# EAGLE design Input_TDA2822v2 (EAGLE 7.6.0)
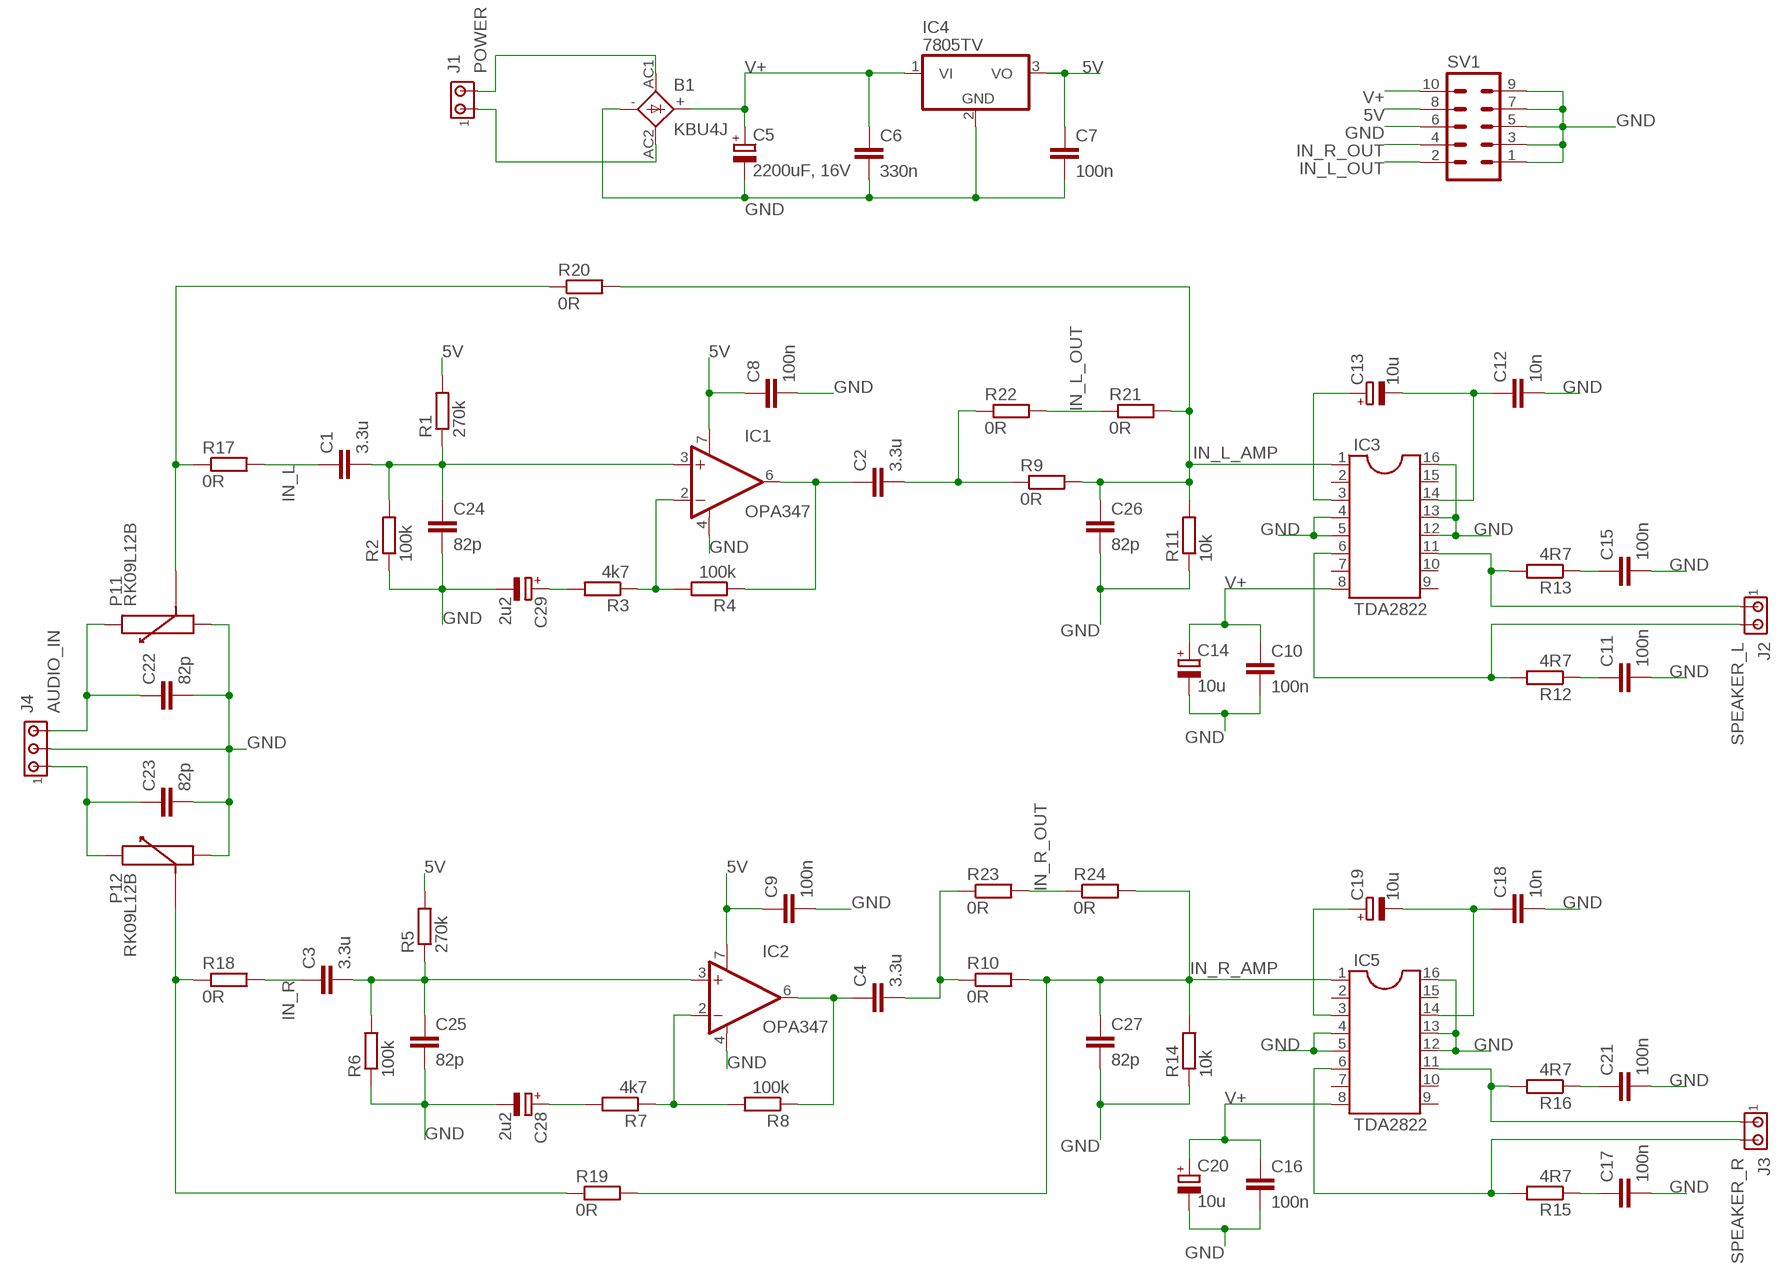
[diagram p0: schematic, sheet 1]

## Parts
B1  KBU4J  KBU  [KBU]
C1  3.3u  C-EU050-055X075  [C050-055X075]
C2  3.3u  C-EU050-055X075  [C050-055X075]
C3  3.3u  C-EU050-055X075  [C050-055X075]
C4  3.3u  C-EU050-055X075  [C050-055X075]
C5  2200uF, 16V  CPOL-EUE5-13  [E5-13]
C6  330n  C-EU050-035X075  [C050-035X075]
C7  100n  C-EU050-025X075  [C050-025X075]
C8  100n  C-EU050-025X075  [C050-025X075]
C9  100n  C-EU050-025X075  [C050-025X075]
C10  100n  C-EU050-025X075  [C050-025X075]
C11  100n  C-EU050-025X075  [C050-025X075]
C12  10n  C-EU025-025X050  [C025-025X050]
C13  10u  CPOL-EUE2-5  [E2-5]
C14  10u  CPOL-EUE2-5  [E2-5]
C15  100n  C-EU050-025X075  [C050-025X075]
C16  100n  C-EU050-025X075  [C050-025X075]
C17  100n  C-EU050-025X075  [C050-025X075]
C18  10n  C-EU025-025X050  [C025-025X050]
C19  10u  CPOL-EUE2-5  [E2-5]
C20  10u  CPOL-EUE2-5  [E2-5]
C21  100n  C-EU050-025X075  [C050-025X075]
C22  82p  C-EU025-024X044  [C025-024X044]
C23  82p  C-EU025-024X044  [C025-024X044]
C24  82p  C-EU025-024X044  [C025-024X044]
C25  82p  C-EU025-024X044  [C025-024X044]
C26  82p  C-EU025-024X044  [C025-024X044]
C27  82p  C-EU025-024X044  [C025-024X044]
C28  2u2  CPOL-EUE2-5  [E2-5]
C29  2u2  CPOL-EUE2-5  [E2-5]
IC1  OPA347  OPA336P  [DIL08]
IC2  OPA347  OPA336P  [DIL08]
IC3  TDA2822  DIL16S  [SOCKET-16]
IC4  7805TV  [TO220V]
IC5  TDA2822  DIL16S  [SOCKET-16]
J1  POWER  350428-1  [350428-1]
J2  SPEAKER_L  350428-1  [350428-1]
J3  SPEAKER_R  350428-1  [350428-1]
J4  AUDIO_IN  350429-1  [350429-1]
P1  RK09L12B  [ALPS-RK09L12B0]
R1  270k  R-EU_0309/V  [0309V]
R2  100k  R-EU_0309/V  [0309V]
R3  4k7  R-EU_0309/V  [0309V]
R4  100k  R-EU_0309/V  [0309V]
R5  270k  R-EU_0309/V  [0309V]
R6  100k  R-EU_0309/V  [0309V]
R7  4k7  R-EU_0309/V  [0309V]
R8  100k  R-EU_0309/V  [0309V]
R9  0R  R-EU_R0603  [R0603]
R10  0R  R-EU_R0603  [R0603]
R11  10k  R-EU_0309/V  [0309V]
R12  4R7  R-EU_0309/V  [0309V]
R13  4R7  R-EU_0309/V  [0309V]
R14  10k  R-EU_0309/V  [0309V]
R15  4R7  R-EU_0309/V  [0309V]
R16  4R7  R-EU_0309/V  [0309V]
R17  0R  R-EU_R0603  [R0603]
R18  0R  R-EU_R0603  [R0603]
R19  0R  R-EU_R0603  [R0603]
R20  0R  R-EU_R0603  [R0603]
R21  0R  R-EU_R0603  [R0603]
R22  0R  R-EU_R0603  [R0603]
R23  0R  R-EU_R0603  [R0603]
R24  0R  R-EU_R0603  [R0603]
SV1  ML10  [ML10]

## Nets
5V: C7.1 C8.1 C9.1 IC1.7(V+) IC2.7(V+) IC4.3(VO) R1.2 R5.2 SV1.8
GND: B1.- C5.- C6.2 C7.2 C8.2 C9.2 C10.2 C11.2 C12.2 C14.- C15.2 C16.2 C17.2 C18.2 C20.- C21.2 C22.2 C23.2 C24.2 C25.2 C26.2 C27.2 C28.- C29.- IC1.4(V-) IC2.4(V-) IC3.4 IC3.5 IC3.12 IC3.13 IC3.16 IC4.2(GND) IC5.4 IC5.5 IC5.12 IC5.13 IC5.16 J4.2 P1.GND1(1:GND$1) P1.GND2(2:GND$1) R2.1 R6.1 R11.1 R14.1 SV1.1 SV1.3 SV1.5 SV1.6 SV1.7 SV1.9
IN_L: C1.1 R17.2
IN_L_AMP: C26.1 IC3.1 R9.2 R11.2 R20.2 R21.2
IN_L_OUT: R21.1 R22.2 SV1.2
IN_R: C3.1 R18.2
IN_R_AMP: C27.1 IC5.1 R10.2 R14.2 R19.2 R24.2
IN_R_OUT: R23.2 R24.1 SV1.4
N$1: C1.2 C24.1 IC1.3(+IN) R1.1 R2.2
N$2: C3.2 C25.1 IC2.3(+IN) R5.1 R6.2
N$3: IC1.2(-IN) R3.1 R4.2
N$4: IC2.2(-IN) R7.1 R8.2
N$5: C2.1 IC1.6(OUT) R4.1
N$6: C4.1 IC2.6(OUT) R8.1
N$7: B1.AC1 J1.2
N$8: B1.AC2 J1.1
N$9: C29.+ R3.2
N$10: IC3.6 J2.2 R12.2
N$11: C28.+ R7.2
N$12: C2.2 R9.1 R22.1
N$13: C4.2 R10.1 R23.1
N$14: C19.+ IC5.3
N$15: C13.+ IC3.3
N$16: C12.1 C13.- IC3.14
N$17: C11.1 R12.1
N$18: C18.1 C19.- IC5.14
N$19: IC5.6 J3.2 R15.2
N$20: C17.1 R15.1
N$21: IC3.11 J2.1 R13.2
N$22: C15.1 R13.1
N$23: IC5.11 J3.1 R16.2
N$24: C21.1 R16.1
N$25: C22.1 J4.3 P1.IN1(1:IN$1)
N$27: C23.1 J4.1 P1.IN2(2:IN$1)
N$28: P1.OUT2(2:OUT$1) R18.1 R19.1
N$29: P1.OUT1(1:OUT$1) R17.1 R20.1
V+: B1.+ C5.+ C6.1 C10.1 C14.+ C16.1 C20.+ IC3.8 IC4.1(VI) IC5.8 SV1.10
Unconnected: IC3.2 IC3.7 IC3.9 IC3.10 IC3.15 IC5.2 IC5.7 IC5.9 IC5.10 IC5.15

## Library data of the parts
B1 = rectifier:KBU: DIOTEC RECTIFIER
C1-C4 C6-C12 C15-C18 C21-C27 = rcl:C-EU: CAPACITOR, European symbol
C5 C13 C14 C19 C20 C28 C29 = rcl:CPOL-EU: POLARIZED CAPACITOR, European symbol
IC1 IC2 = burr-brown:OPA336: CMOS Operational Amplifiers Single-Supply, MicroPower, MicroAmplifier(TM) Series; OC_FARNELL: unknown; OC_NEWARK: unknown
IC3 IC5 = ic-package:DIL16: Dual In Line / Socket
IC4 = linear:78*: Positive VOLTAGE REGULATOR Source: http://cache.national.com/ds/LM/LM78L05.pdf http://www.fairchildsemi.com/ds/LM/LM7805.pdf
J1-J3 = con-amp:350428-1: Universal MATE-N-LOK .250" Centerline, 600 V, 19 - 36 A max
J4 = con-amp:350429-1: Universal MATE-N-LOK .250" Centerline, 600 V, 19 - 36 A max Source: http://catalog.tycoelectronics.com/ .. ENG_CD_350429_Y.pdf
P1 = my:RK09L12B
R1-R24 = rcl:R-EU_: RESISTOR, European symbol
SV1 = con-ml:ML10: HARTING; OC_FARNELL: unknown; OC_NEWARK: unknown

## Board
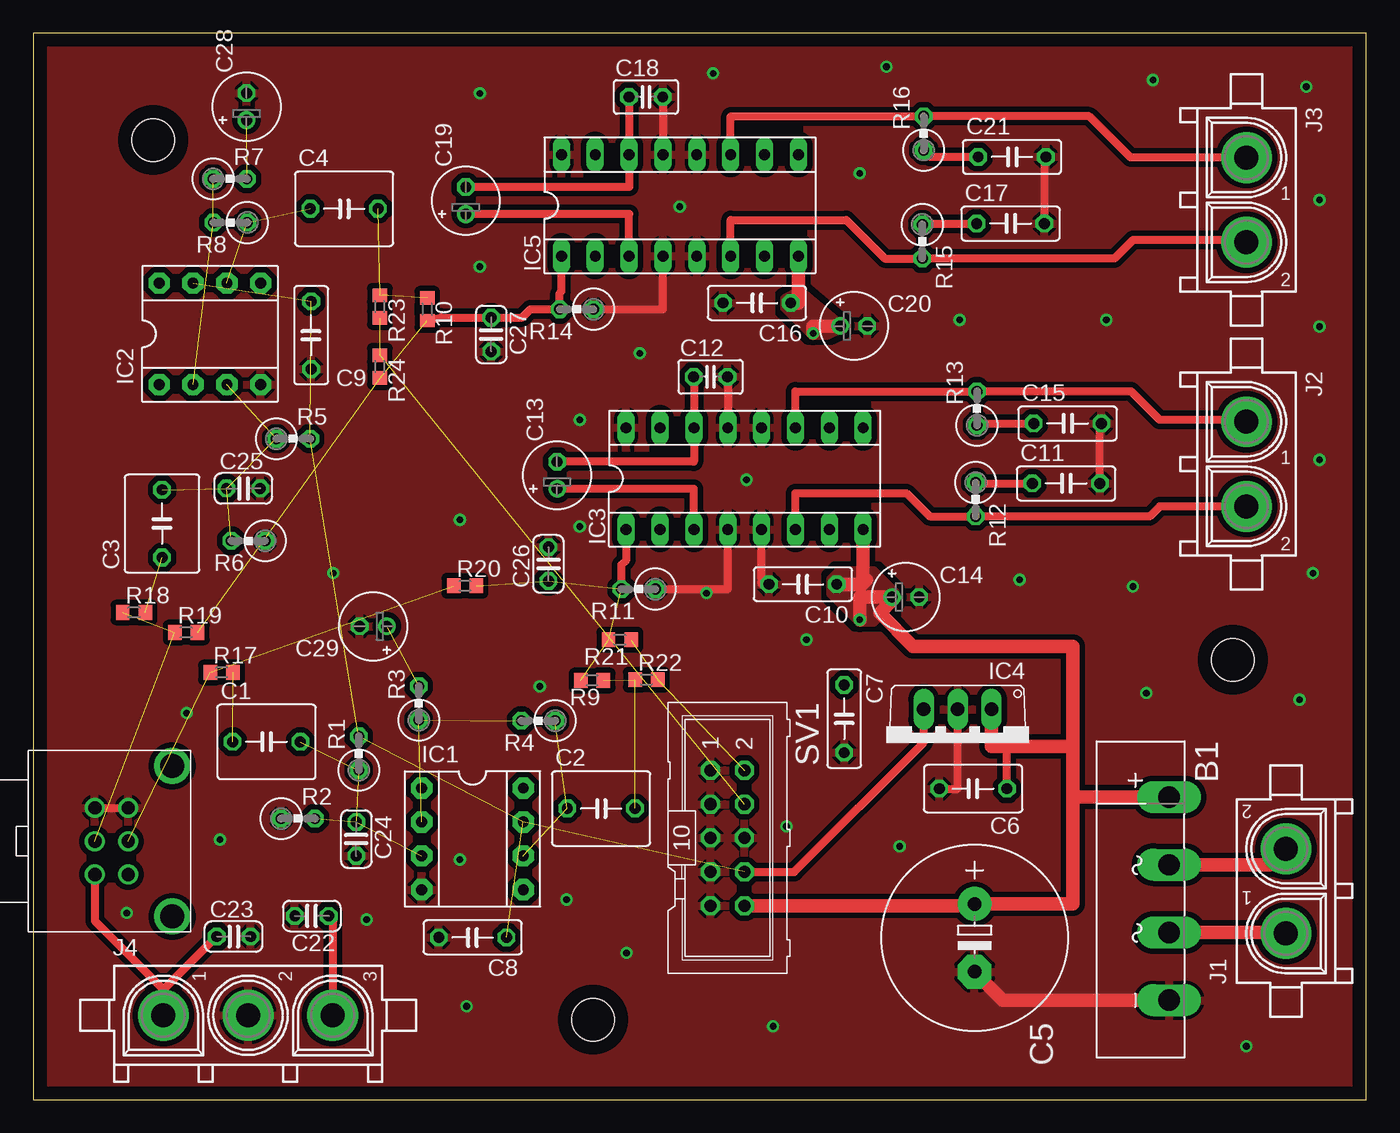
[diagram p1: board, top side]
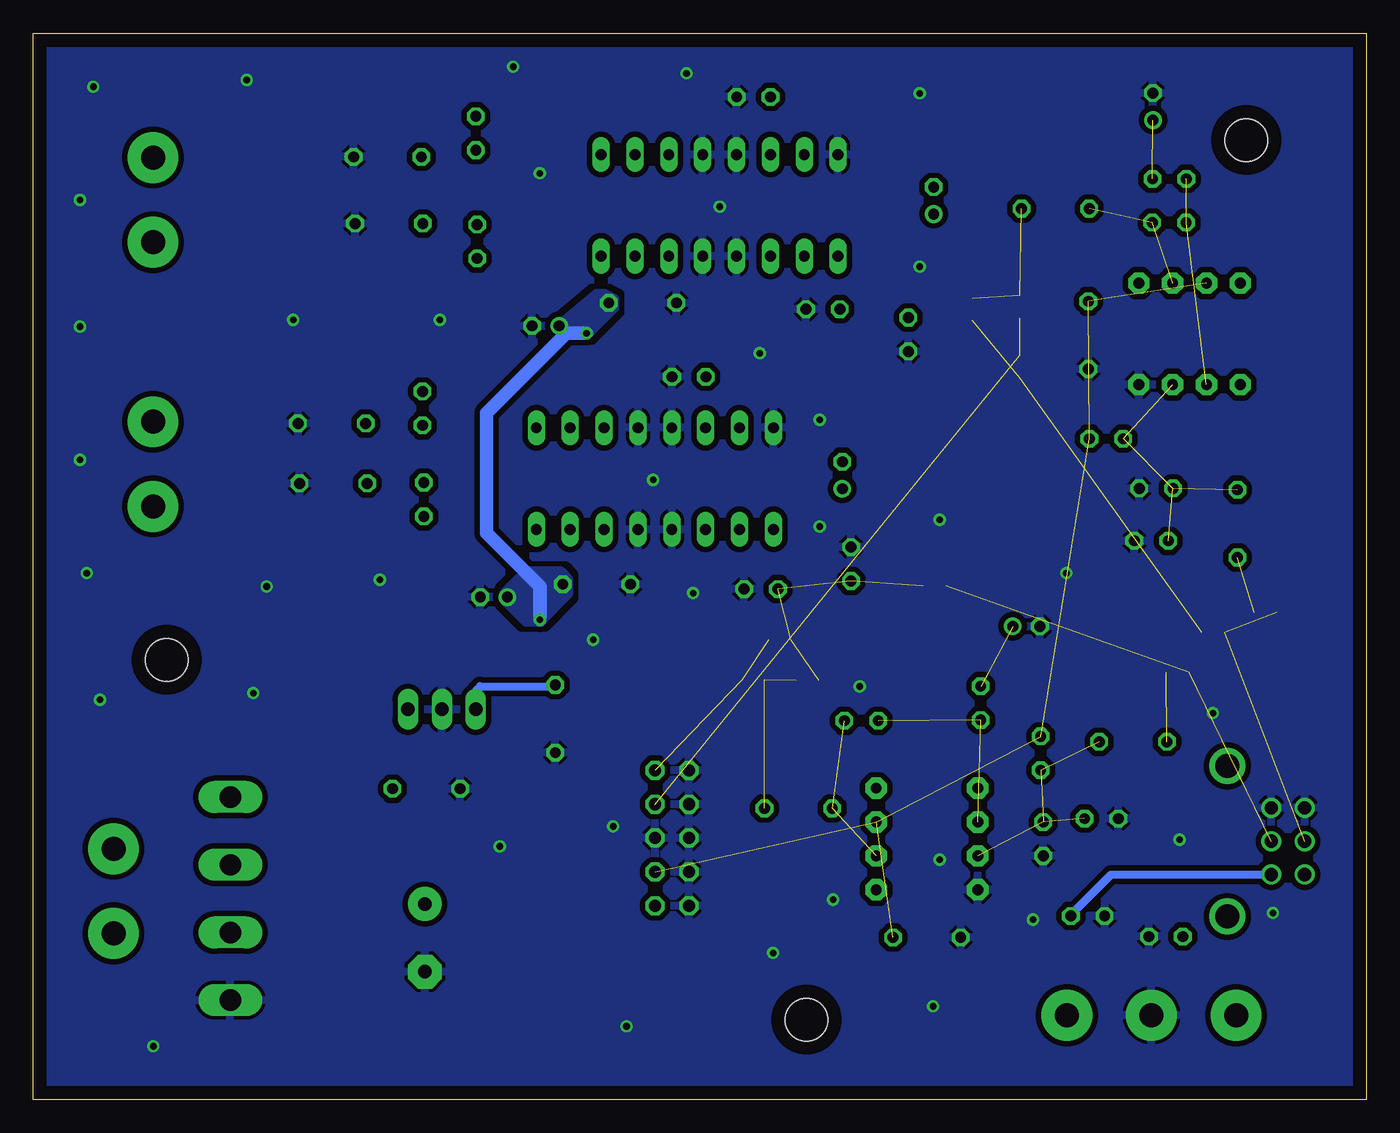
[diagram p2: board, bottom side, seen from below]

Size 100 x 80 mm. Coordinates in mm from the lower left corner, seen from the top.
Outline: 0,0 100,0 100,80 0,80 0,0
Copper layers (1*16): Top 0.035mm / dielectric 1.5mm / Bottom 0.035mm
Design rules "default": minimum track width 10mil, minimum drill 24mil, track to track 8mil, track to pad 8mil, pad to pad 8mil, via to via 8mil, smd to smd 8mil, copper to edge 40mil, drill to drill 8mil, minimum pad ring 10mil, minimum via ring 8mil, stop-mask expansion 4mil, vias tented up to drill 0mil, thermal gap 10mil
Holes 3.2 mm at 9,72 90,33 42,6

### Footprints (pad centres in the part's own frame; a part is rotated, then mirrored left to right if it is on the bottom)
KBU = drill 1.6 long: + -7.62,2.54; - 7.62,2.54; AC1 -2.54,2.54; AC2 2.54,2.54
C050-055X075 = drill 0.813 octagon: 1 -2.54,0; 2 2.54,0
E5-13 = drill 1.016 pad 2.54: + -2.54,0 | drill 1.016 pad 2.54 octagon: - 2.54,0
C050-035X075 = drill 0.813 octagon: 1 -2.54,0; 2 2.54,0
C050-025X075 = drill 0.813 octagon: 1 -2.54,0; 2 2.54,0
C025-025X050 = drill 0.813 octagon: 1 -1.27,0; 2 1.27,0
E2-5 = drill 0.813 pad 1.27: + -1.016,0 | drill 0.813 pad 1.27 octagon: - 1.016,0
C025-024X044 = drill 0.813 octagon: 1 -1.27,0; 2 1.27,0
DIL08 = drill 0.813 pad 1.6 octagon: 1 -3.81,-3.81; 2 -1.27,-3.81; 3 1.27,-3.81; 4 3.81,-3.81; 5 3.81,3.81; 6 1.27,3.81; 7 -1.27,3.81; 8 -3.81,3.81
SOCKET-16 = drill 0.813 long: 1 -8.89,-3.81; 2 -6.35,-3.81; 3 -3.81,-3.81; 4 -1.27,-3.81; 5 1.27,-3.81; 6 3.81,-3.81; 7 6.35,-3.81; 8 8.89,-3.81; 9 8.89,3.81; 10 6.35,3.81; 11 3.81,3.81; 12 1.27,3.81; 13 -1.27,3.81; 14 -3.81,3.81; 15 -6.35,3.81; 16 -8.89,3.81
TO220V = drill 1.016 long: 1 -2.54,-2.54; 2 0,-2.54; 3 2.54,-2.54
350428-1 = drill 1.8 pad 3.81: 1 -3.175,0; 2 3.175,0
350429-1 = drill 1.8 pad 3.81: 1 -6.35,0; 2 0,0; 3 6.35,0
ALPS-RK09L12B0 = drill 1: GND1 3.3,-2.5; GND2 5.8,-2.5; IN1 3.3,2.5; IN2 5.8,2.5; OUT1 3.3,0; OUT2 5.8,0 | drill 1.8: P$1 0,5.65; P$2 0,-5.65
0309V = drill 0.813 octagon: 1 -1.27,0; 2 1.27,0
R0603 = smd 1 x 1.1: 1 -0.85,0; 2 0.85,0
ML10 = drill 0.914 octagon: 1 -5.08,-1.27; 2 -5.08,1.27; 3 -2.54,-1.27; 4 -2.54,1.27; 5 0,-1.27; 6 0,1.27; 7 2.54,-1.27; 8 2.54,1.27; 9 5.08,-1.27; 10 5.08,1.27

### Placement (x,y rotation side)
B1  82.68,15.07 270 top
C1  17.49,26.84 0 top
C2  42.6,21.84 0 top
C3  9.66,43.21 90 top
C4  23.32,66.84 0 top
C5  70.62,12.13 270 top
C6  70.51,23.32 180 top
C7  60.84,28.57 270 top
C8  32.96,12.16 180 top
C9  20.84,57.35 270 top
C10  57.74,38.66 180 top
C11  77.49,46.23 0 top
C12  50.81,54.23 0 top
C13  39.3,46.84 90 top
C14  65.45,37.7 0 top
C15  77.6,50.73 0 top
C16  54.29,59.77 180 top
C17  73.32,65.73 0 top
C18  45.96,75.23 0 top
C19  32.45,67.45 90 top
C20  61.56,58.05 0 top
C21  73.43,70.73 0 top
C22  20.89,13.77 180 top
C23  15.03,12.23 0 top
C24  24.23,19.55 270 top
C25  15.76,45.85 0 top
C26  38.65,40.18 90 top
C27  34.35,57.4 270 top
C28  16,74.5 90 top
C29  25.5,35.5 180 top
IC1  32.95,19.55 270 top
IC2  13.25,57.45 0 top
IC3  53.37,46.59 0 top
IC4  69.35,26.74 180 top
IC5  48.51,67.09 0 top
J1  93.98,15.64 90 top
J2  91.02,47.68 270 top
J3  91.02,67.5 270 top
J4  16.11,6.32 0 top
P1  10.42,19.38 180 top
R1  24.42,25.98 90 top
R2  19.86,21.08 0 top
R3  28.92,29.74 90 top
R4  37.88,28.42 180 top
R5  19.5,49.58 0 top
R6  16.12,41.92 180 top
R7  14.76,69.08 0 top
R8  14.78,65.8 180 top
R9  41.92,31.45 180 top
R10  29.55,59.29 270 top
R11  45.4,38.3 180 top
R12  70.7,45.02 270 top
R13  70.8,51.86 90 top
R14  40.76,59.3 180 top
R15  66.7,64.38 270 top
R16  66.8,72.5 90 top
R17  14.13,32.05 0 top
R18  7.55,36.55 0 top
R19  11.47,35.05 0 top
R20  32.39,38.55 0 top
R21  44,34.5 180 top
R22  46,31.5 0 top
R23  26,59.5 270 top
R24  26,55 270 top
SV1  52.08,19.62 270 top

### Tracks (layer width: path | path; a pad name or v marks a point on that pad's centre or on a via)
5V  (6 unrouted)
  Top 0.61: SV1.8 57.08,17.08 66.81,26.81 IC4.3
  Bottom 0.61: IC4.3 66.81,30.69 66.5,31 60.45,31 C7.1
GND  (via drill 0.5)
  Top 0.61: J4.2 16.3,6.51 | P1.GND2 P1.GND1 | C10.2 54.64,38.66 IC3.5 | C11.2 80.03,50.73 C15.2 | C18.2 IC5.13 | C12.2 52.1,54.23 IC3.13 | R11.1 52.1,38.3 IC3.4 | R14.1 47.24,59.3 IC5.4 | C21.2 75.86,70.62 C17.2 | C6.2 69.35,23.32 IC4.2
  Top 1.016: B1.- 72.76,7.45 C5.-
  other vias: 45.5,56 48.5,67 51,77 62,69.5 84,76.5 80.5,58.5 69.5,58.5 82.5,38.5 74,39 83.5,30.5 50.5,38 38,31 40,15 22.5,39.5 11.5,29 33.5,62.5 41,51 32,43.5 41,43 44.5,11 32,18 25,13.5 14,19.5 7,14 32.5,7 55.5,5.5 91,4 95,30 65,19 58,34.5 56.5,20.5 64,77.5 96.5,58 95.5,76 96,39.5 96.5,48 96.5,67.5 33.5,75.5 53.5,46.5
  pour Top (isolate 0.406, rank 2): 0.5,79.5 0.5,0.5 99.5,0.5 99.5,79.5
  pour Bottom (isolate 0.406, rank 2): 0.5,79.5 0.5,0.5 99.5,0.5 99.5,79.5
IN_L  (1 unrouted)
IN_L_AMP  (4 unrouted)
  Top 0.61: R11.2 44.13,40.13 44.5,40.5 44.5,42.76 IC3.1
IN_L_OUT  (2 unrouted)
IN_R  (1 unrouted)
IN_R_AMP  (2 unrouted)
  Top 0.61: IC5.1 39.62,60.62 39.49,60.49 R14.2 37.3,59.3 36.67,58.67 C27.1 30.56,58.67 R10.2
IN_R_OUT  (2 unrouted)
N$1  (4 unrouted)
N$2  (4 unrouted)
N$3  (2 unrouted)
N$4  (2 unrouted)
N$5  (2 unrouted)
N$6  (2 unrouted)
N$7
  Top 1.016: J1.2 92.78,17.61 B1.AC1
N$8
  Top 1.016: J1.1 93.92,12.53 B1.AC2
N$9  (1 unrouted)
N$10
  Top 0.61: IC3.6 57.18,45.5 65.5,45.5 67.25,43.75 R12.2 83.75,43.75 84.5,44.5 J2.2
N$11  (1 unrouted)
N$12  (2 unrouted)
N$13  (2 unrouted)
N$14
  Top 0.61: IC5.3 44.7,66.43 C19.+
N$15
  Top 0.61: IC3.3 49.56,45.82 C13.+
N$16
  Top 0.61: C12.1 49.56,54.23 IC3.14 49.56,47.86 C13.-
N$17
  Top 0.61: R12.1 70.7,46.23 C11.1
N$18
  Top 0.61: C18.1 IC5.14 44.7,68.47 C19.-
N$19
  Top 0.61: J3.2 90.84,64.5 82.5,64.5 81.11,63.11 R15.2 63.89,63.11 61,66 52.32,66 IC5.6
N$20
  Top 0.61: R15.1 66.78,65.73 C17.1
N$21
  Top 0.61: J2.1 90.88,51 84.5,51 82.37,53.13 R13.2 57.18,53.13 IC3.11
N$22
  Top 0.61: R13.1 70.8,50.73 C15.1
N$23
  Top 0.61: IC5.11 52.32,73.77 R16.2 79.23,73.77 82.33,70.67 J3.1
N$24
  Top 0.61: R16.1 67.3,70.73 C21.1
N$25
  Top 0.61: J4.3 22.5,6.36 22.5,13.43 C22.1
  Bottom 0.61: C22.1 22.16,13.84 19.12,16.88 P1.IN1
N$27
  Top 0.61: 9.76,8.26 J4.1 | P1.IN2 4.62,13.4 9.76,8.26 | 9.76,8.26 9.79,8.26 C23.1
N$28  (2 unrouted)
N$29  (2 unrouted)
V+  (via drill 0.5)
  Top 0.61: C6.1 73.05,26.5 74.5,26.5
  Top 1.016: B1.+ 78,22.69 | 78,22.69 78,26.5 | 78,26.5 74.5,26.5 71.89,26.5 IC4.1 | 78,22.69 78,14.67 C5.+ 70.62,14.54 SV1.10 | C20.+ 58.5,58.05 v58.5,57.5 | v62,36 62,37.7 C14.+ 64.43,37.43 63.5,36.5 66,34 78,34 78,26.5 | IC3.8 62.26,39.24 62.5,39 62.16,38.66 C10.1 | IC5.8 57.4,59.77 C16.1
  Bottom 1.016: v62,36 62,38.5 66,42.5 66,51.5 60,57.5 v58.5,57.5
  pour Top (isolate 0.406, no thermals): 58.5,57.5 56.5,59.5 56.5,60 57.5,60.5 60.5,58 59.5,57.5
  pour Bottom (isolate 0.406, no thermals): 58.5,57.5 56.5,59.5 56.5,60 57.5,60.5 60.5,58 59.5,57.5
  pour Bottom (isolate 0.406, no thermals): 62,36 60,38 60,38.5 60,39 60.5,39.5 63,39.5 64.5,38 64.5,37.5 63,36
  pour Top (isolate 0.406, no thermals): 62,36 60,38 60,38.5 60,39 60.5,39.5 63,39.5 64.5,38 64.5,37.5 63,36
